TYPE iState_Enum :
(
	iState_Prepare			:= 0,
	iState_Connect			:= 1,
	iState_GetNameSpaceIndex:= 2,
	iState_GetNodeHandle	:= 3,
	iState_Read				:= 4,
	iState_ReleaseHandle	:= 5,
	iState_Disconnect		:= 6,
	iState_Error			:= 7
);
END_TYPE
